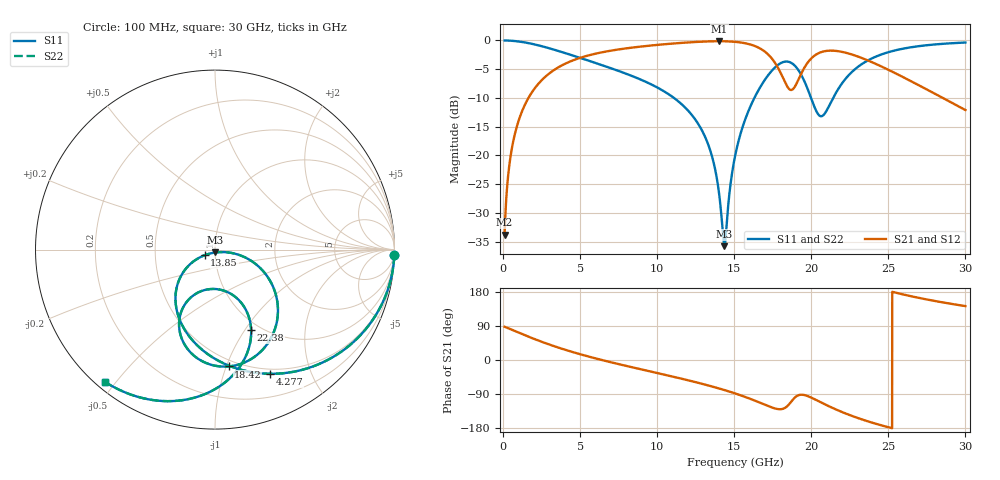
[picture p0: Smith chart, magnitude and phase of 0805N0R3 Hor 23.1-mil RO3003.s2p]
# GHz S MA R 50
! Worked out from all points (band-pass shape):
!   3201 points, 100 MHz to 30 GHz, reference 50 ohm
!   highest |S21| = -0.14 dB at 14.02 GHz (marker M1); lowest = -33.8 dB at 100 MHz (marker M2)
!   |S21| within 3 dB of the highest: 4.874 GHz to 17.44 GHz (12.57 GHz wide, 113 % of centre); 19.99 GHz to 23.36 GHz (3.365 GHz wide, 15.5 % of centre)
!   lowest |S11| = -35.8 dB at 14.37 GHz (marker M3), VSWR 1.03, Z = 50.2 - j1.62 ohm
!   |S11| at or under -10 dB: 11.09 GHz to 16.31 GHz (5.215 GHz wide, 38.1 % of centre); 19.99 GHz to 21.42 GHz (1.435 GHz wide, 6.93 % of centre)
!   |S22| runs from -35.8 to 0.0 dB; largest |S21 - S12| = 0
!   S11 on the Smith chart (normalised r, x): 100 MHz: 1, -65; 4.277 GHz: 0.45, -1.45; 13.85 GHz: 0.89, -0.06; 18.42 GHz: 0.45, -1.02; 22.38 GHz: 0.91, -1.07; 30 GHz: 0.03, -0.47
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0.1  0.9996 -1.8  0.02047 87.8  0.02047 87.8  0.9996 -1.8
0.5204688  0.9941 -9.2  0.1052 80.7  0.1052 80.7  0.9941 -9.2
1.230594  0.9698 -21.4  0.2422 68.5  0.2422 68.5  0.9698 -21.4
2.669531  0.8796 -44.2  0.4738 45.6  0.4738 45.6  0.8796 -44.2
4.276656  0.7579 -65.9  0.6496 23.9  0.6496 23.9  0.7579 -65.9
5.089563  0.6989 -75.5  0.7121 14.2  0.7121 14.2  0.6989 -75.5
7.472219  0.5446 -100.2  0.8344 -10.6  0.8344 -10.6  0.5446 -100.2
10.06978  0.386 -124.1  0.9164 -35.0  0.9164 -35.0  0.386 -124.1
12.60194  0.1938 -146.8  0.9714 -59.5  0.9714 -59.5  0.1938 -146.8
13.854  0.06533 -151.4  0.9842 -73.2  0.9842 -73.2  0.06533 -151.4
14.02219  0.04615 -147.3  0.9844 -75.2  0.9844 -75.2  0.04615 -147.3
14.36791  0.01629 -80.8  0.9832 -79.3  0.9832 -79.3  0.01629 -80.8
15.05  0.09822 -11.4  0.9724 -88.1  0.9724 -88.1  0.09822 -11.4
15.89094  0.2378 -19.3  0.9337 -100.2  0.9337 -100.2  0.2378 -19.3
17.16169  0.4907 -44.4  0.7642 -120.9  0.7642 -120.9  0.4907 -44.4
18.42309  0.6553 -83.4  0.4013 -122.5  0.4013 -122.5  0.6553 -83.4
19.24534  0.5308 -110.4  0.4814 -92.0  0.4814 -92.0  0.5308 -110.4
20.03956  0.3022 -117.1  0.7065 -100.0  0.7065 -100.0  0.3022 -117.1
20.74969  0.2222 -85.1  0.7995 -114.3  0.7995 -114.3  0.2222 -85.1
22.3755  0.4901 -65.7  0.773 -143.5  0.773 -143.5  0.4901 -65.7
25.01978  0.7917 -91.8  0.5543 -177.6  0.5543 -177.6  0.7917 -91.8
30  0.9588 -129.9  0.2484 142.2  0.2484 142.2  0.9588 -129.9
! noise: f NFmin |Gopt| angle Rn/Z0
0.1  0.01508  0.9958  0.6256  0.8184
3.417  0.00855  0.78  23.05  0.007652
6.743  0.01313  0.7274  41.72  0.008392
10.06  0.01843  0.7197  58.96  0.009949
13.39  0.02819  0.7593  74.85  0.01513
16.7  0.08325  0.8947  90.16  0.08625
20.03  0.1963  0.9467  105  0.3061
23.35  0.111  0.896  118.5  0.06143
26.67  0.1145  0.8887  131  0.03914
30  0.1395  0.9006  143  0.03172
